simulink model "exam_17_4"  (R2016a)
settings: Solver=ode15s  StartTime=0  StopTime=1  RelTol=1e-3
libraries: powerlib x4

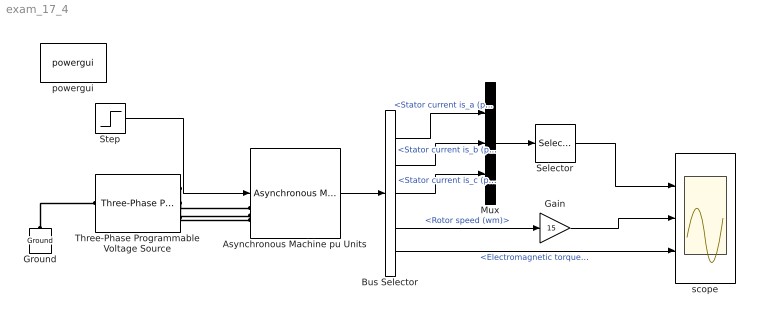
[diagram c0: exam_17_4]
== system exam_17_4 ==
  Asynchronous Machine pu Units : powerlib/Machines/Asynchronous Machine pu Units  RotorType=Squirrel-cage  PresetModel=No  MechanicalLoad=Torque Tm  ShowDetailedParameters=on  ReferenceFrame=Rotor  Units=pu  MeasurementBus=off  NominalParameters=[10000 380 50]  Stator=[0.458 2.578e-03]  Rotor=[0.349 0.333e-02]  Cage1=[0.01909 0.0397]  Cage2=[0.01909 0.0397]  Lm=0.088  Mechanical=[0.6 0.0 2]  PolePairs=2  InitialConditions="[ 1,0   0,0,0   0,0,0 ]"  SimulateSaturation=off  Saturation="[0.212,0.4201,0.8125,1.0979,1.4799,2.2457,3.2586,4.5763,6.4763 ;   0.5,0.7,0.9,1,1.1,1.2 ,1.3,1.4,1.5]"  LoadFlowParameters=0  TsPowergui=0  TsBlock=-1  IterativeModel=Trapezoidal non iterative  IterativeDiscreteModel=Trapezoidal non iterative  Pmec=0
  Bus Selector : BusSelector  OutputSignals=Stator measurements.Stator current is_a (pu),Stator measurements.Stator current is_b (pu),Stator measurements.Stator current is_c (pu),Mechanical.Rotor speed (wm),Mechanical.Electromagnetic torque Te (pu)
  Gain : Gain  Gain=15
  Ground : powerlib/Elements/Ground  LConnTagsString=a
  Mux : Mux  Inputs=3
  Selector : Selector  IndexMode=Zero-based  InputPortWidth=3  IndexOptions=Index vector (dialog)  Indices=[0]  OutputSizes=1
  Step : Step  Time=0.2  Before=67.7642  After=100  SampleTime=0.001  VectorParams1D=off  ZeroCross=off
  Three-Phase Programmable Voltage Source : powerlib/Electrical Sources/Three-Phase Programmable Voltage Source  PositiveSequence="[460  0 50]"  VariationEntity=None  VariationType=Table of time-amplitude pairs  VariationTypeAlt=Step  VariationStep=0.5  VariationRate=10  VariationMagnitude=0.3  VariationFrequency=2  VariationTiming=[1 2]  VariationPhaseA=off  Amplitudes=[1 0.8 1.2 1.0]  TimeValues=[0 0.1 0.15 0.2]  HarmonicGeneration=off  HarmonicA=[3 0.2 -25 0]  HarmonicB=[2 0.15 35 2]  Timing="[0.05  3]"  BusType=swing  Pref=0  Qref=0  Qmin=-inf  Qmax=inf
  powergui : powerlib/powergui  Priority=1  SimulationMode=Continuous  SolverType=Tustin/Backward Euler (TBE)  SampleTime=50e-6  frequency=60  SPID=off  DisableSnubberDevices=off  DisableRonSwitches=off  DisableVfSwitches=off  SwTol=0  DisplayEquations=off  Interpol=off  ExternalGateDelay=off  methode=off  Ts=10  FunctionMessages=off  echomessages=off  HookPort=off  EnableUseOfTLC=off  x0status=blocks  frequencyindice=50  Pbase=50e6  ErrMax=1e-4  Iterations=50  UnitsV=kV  UnitsW=MW  buscounter=0  RestoreLinks=warning  ResistiveCurrentMeasurement=off  Frange=[0:2:500]  Ylog=off  Xlog=on  ShowGrid=off  save=off  variable=ZData  structure=0  ZoomFFT=off  StartTime=0.0  cycles=1  DisplayStyle=1  fundamental=60  FreqAxis=off  MaxFrequency=1000  frequencyindicesteady=1  RmsSteady=1  display=off
  scope : Scope  NumInputPorts=3
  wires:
  Asynchronous Machine pu Units/1 -> Bus Selector/1
  Step/1 -> Asynchronous Machine pu Units/1
  Bus Selector/1 -> Mux/1  "<Stator current is_a (pu)>"
  Bus Selector/2 -> Mux/2  "<Stator current is_b (pu)>"
  Bus Selector/3 -> Mux/3  "<Stator current is_c (pu)>"
  Mux/1 -> Selector/1
  Selector/1 -> scope/1
  Bus Selector/4 -> Gain/1  "<Rotor speed (wm)>"
  Gain/1 -> scope/2
  Bus Selector/5 -> scope/3  "<Electromagnetic torque Te (pu)>"
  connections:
  Ground/LConn1 -- Three-Phase Programmable Voltage Source/LConn1
  Three-Phase Programmable Voltage Source/RConn1 -- Asynchronous Machine pu Units/LConn1
  Three-Phase Programmable Voltage Source/RConn2 -- Asynchronous Machine pu Units/LConn2
  Three-Phase Programmable Voltage Source/RConn3 -- Asynchronous Machine pu Units/LConn3
